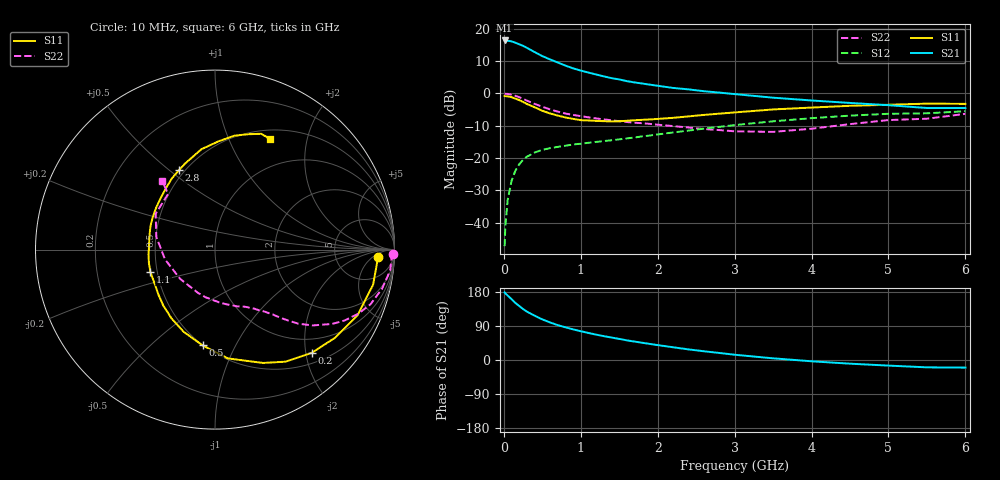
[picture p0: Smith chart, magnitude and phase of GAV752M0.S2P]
! Infineon Technologies  Discrete & RF Semiconductors
! BF775
! Si NPN RF Bipolar Junction Transistor in SOT23
! VCE = 0.75 V  IC = 2 mA
! Common Emitter S-Parameters:  May  1996
# GHz  S  MA  R  50
!  f  S11  S21  S12  S22
! GHz  MAG  ANG  MAG  ANG  MAG  ANG  MAG  ANG
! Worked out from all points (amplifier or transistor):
!   36 points, 10 MHz to 6 GHz, reference 50 ohm
!   highest |S21| = 16.4 dB at 10 MHz (marker M1)
!   |S21| within 3 dB of that: start of sweep to 354.4 MHz
!   unconditionally stable (mu >= 1): 1.051 GHz to end of sweep
!   at 250 MHz: K = 0.30, MSG = 17.7 dB, |S12| = -20.6 dB
!   at 1.4 GHz: K = 1.17, MAG = 7.1 dB, |S12| = -14.5 dB
!   at 6 GHz: K = 1.07, MAG = -1.2 dB, |S12| = -5.5 dB
!   S11 on the Smith chart (normalised r, x): 10 MHz: 17, -8; 200 MHz: 0.70, -2.12; 500 MHz: 0.50, -0.75; 1.1 GHz: 0.46, -0.13; 2.8 GHz: 0.47, +0.54; 6 GHz: 0.61, +1.43
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0.01  0.9097 -2.5  6.613 178.4  0.0043 85.0  0.9939 -1.3
0.02  0.9055 -5.0  6.608 175.8  0.0089 87.1  0.9848 -2.7
0.05  0.9023 -12.5  6.539 170.1  0.0225 82.2  0.983 -6.8
0.1  0.8741 -24.8  6.403 160.5  0.0442 76.0  0.9559 -13.2
0.15  0.8293 -36.4  6.101 150.6  0.0636 68.8  0.9181 -19.4
0.2  0.7881 -46.9  5.776 142.5  0.0797 63.4  0.8736 -24.2
0.25  0.7378 -57.8  5.459 134.5  0.0934 58.1  0.8228 -28.7
0.3  0.6861 -67.0  5.082 127.6  0.1046 54.1  0.773 -32.4
0.4  0.6107 -83.2  4.371 117.0  0.1214 47.9  0.6893 -37.8
0.5  0.538 -97.4  3.783 107.1  0.1336 43.4  0.6221 -41.6
0.6  0.49 -110.9  3.368 99.1  0.1419 40.8  0.5659 -44.2
0.7  0.4535 -122.3  3.012 92.1  0.1485 38.9  0.5223 -46.4
0.9  0.4032 -141.3  2.447 80.9  0.1616 36.7  0.4642 -49.7
1.1  0.381 -160.9  2.102 71.3  0.1718 36.2  0.4262 -53.0
1.3  0.3715 -175.6  1.835 63.0  0.1828 36.4  0.3954 -56.3
1.6  0.3769 164.2  1.549 51.8  0.201 37.2  0.3603 -62.2
2.2  0.4182 136.1  1.216 33.6  0.2483 37.1  0.3119 -78.0
2.8  0.4855 114.5  1.03 18.6  0.3033 34.2  0.2704 -101.5
3.5  0.5644 97.7  0.859 4.4  0.3696 27.5  0.2536 -140.0
4.5  0.6429 80.5  0.712 -9.7  0.4528 15.4  0.3344 167.8
5.5  0.6946 68.3  0.594 -19.4  0.4916 1.5  0.4053 130.1
6  0.6889 63.5  0.594 -20.1  0.53 -2.3  0.4824 127.6
